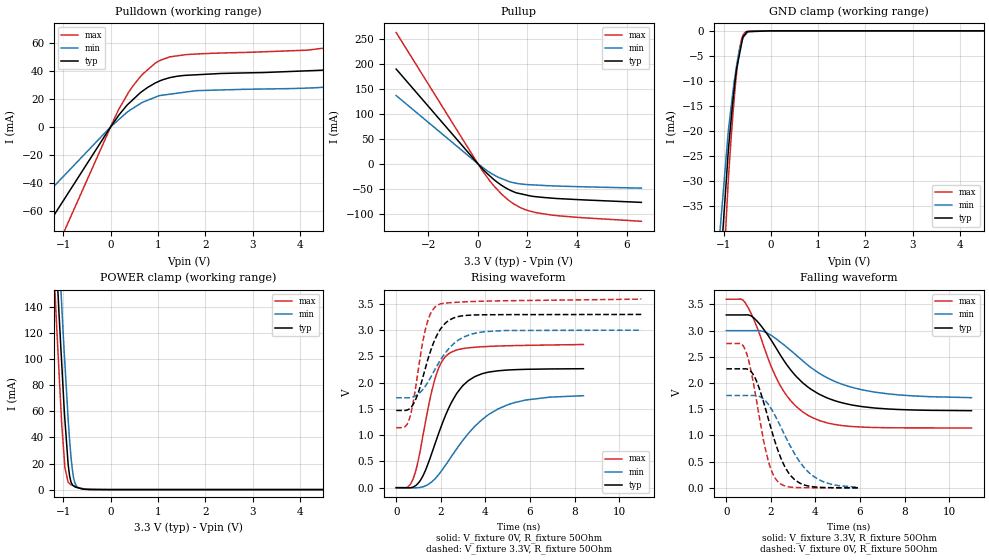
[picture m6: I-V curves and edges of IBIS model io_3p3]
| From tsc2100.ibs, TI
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|   io_3p3 Model
[Model]   io_3p3
Model_type   I/O
Polarity   Non-Inverting
Enable   Active-Low
Vinl = 0.99
Vinh = 2.31
Vmeas = 1.65
Vref = 1.65
Cref = 10pF
Rref = 50
|   typ   min   max
|   (nom PVT)   (fast PVT)   (slow PVT)
|C_comp from frequency sweep method (F=13MHz)
|Average
|C_comp   2.863e-12   2.648e-12   3.065e-12
|ON state : BUFFER OUTPUT TURNED HIGH
|C_comp   4.084e-12   3.666e-12   4.474e-12
|OFF state: BUFFER IN HIGH IMPEDANCE
|C_comp   1.642e-12   1.629e-12   1.656e-12
|C_comp from LC tank measurement(L=1nH)
|Average
|Resonant Frequency(Hz)   4.310e+09   4.340e+09   4.270e+09
C_comp   1.373e-12   1.353e-12   1.400e-12
|ON state : BUFFER OUTPUT TURNED HIGH
|Resonant Frequency(Hz)   4.130e+09   4.170e+09   4.070e+09
|C_comp   1.487e-12   1.458e-12   1.531e-12
|OFF state: BUFFER IN HIGH IMPEDANCE
|Resonant Frequency(Hz)   4.490e+09   4.510e+09   4.470e+09
|C_comp   1.258e-12   1.247e-12   1.269e-12
| Where nom  PVT is Nominal Process, 3.3V, 26C
|   Fast PVT is Strong Process,  3.6V, -40C
|   Slow PVT is Weak Process,   3V, 86C
[Model Spec]
|Subparameter   typ   min   max
Vinh   2.31   2.1   2.52
Vinl   0.99   0.9   1.08
[Voltage Range]   3.3   3   3.6
|Ambient Temperature   25   85   -40
|Junction Temperature
[Temperature Range]   26   86   -40
[Pullup Reference]   3.3   3   3.6
[Pulldown Reference]   0   0   0
[Power Clamp Reference]   3.3   3   3.6
[GND Clamp Reference]   0   0   0
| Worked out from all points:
|   slope of the pulldown table from 0 to 0.495 V, typ, clamps not added: 24.4 ohm
|   slope of the pullup table from 0 to 0.495 V, typ, clamps not added: 19.8 ohm
|   GND clamp passes 1 mA (typ) near -0.57 V on its own axis
|   POWER clamp passes 1 mA (typ) near -0.64 V on its own axis
|   falling waveform, V_fixture 3.3V, R_fixture 50Ohm: 20-80 % time 2.13ns typ, 2.66ns min, 1.62ns max; typ from 3.3 V to 1.47 V
|   rising waveform, V_fixture 0V, R_fixture 50Ohm: 20-80 % time 1.32ns typ, 2.09ns min, 821ps max; typ from 0 V to 2.27 V
|   rising waveform, V_fixture 3.3V, R_fixture 50Ohm: 20-80 % time 853ps typ, 1.22ns min, 597ps max; typ from 1.47 V to 3.3 V
|   falling waveform, V_fixture 0V, R_fixture 50Ohm: 20-80 % time 1.03ns typ, 1.4ns min, 738ps max; typ from 2.27 V to 0.001 V
[Pulldown]
|   Voltage   I(typ)   I(min)   I(max)
-3.3V     -174.4mA   -117.2mA   -251.9mA
-3mV      -158.6uA   -106.5uA   -229uA
172.8mV   8.404mA    5.266mA    12.6mA
478.8mV   19.78mA    13.48mA    29.65mA
684mV     25.89mA    17.74mA    38.01mA
1.026V    32.75mA    22.4mA     47.35mA
1.591V    36.96mA    24.99mA    51.77mA
4.162V    40.2mA     27.84mA    54.99mA
5.141V    44.75mA    31.56mA    62.91mA
5.666V    52.18mA    36.03mA    74.45mA
6.154V    64.13mA    43.44mA    92.9mA
6.6V      80.76mA    50.23mA    118mA
[GND Clamp]
|   Voltage   I(typ)   I(min)   I(max)
-3.3V     -1.799A    -1.622A    -1.991A
-1.505V   -108.3mA   -89.01mA   -138.1mA
-897.6mV  -23.79mA   -19.91mA   -29.58mA
-792mV    -13.12mA   -11.42mA   -15.51mA
-726mV    -7.734mA   -7.055mA   -8.618mA
-702mV    -6.579mA   -5.702mA   -6.431mA
-658.8mV  -4.5mA     -3.681mA   -3.454mA
-622.8mV  -2.767mA   -2.351mA   -1.787mA
-590.7mV  -1.223mA   -1.433mA   -927.5uA
-532.8mV  -520.6uA   -757.3uA   -190.4uA
-285mV    -102.3uA   -1.16uA    -4.272uA
6.6V      0A         0A         0A
[Pullup]
|   Voltage   I(typ)   I(min)   I(max)
-3.3V     189.3mA    136.3mA    262.3mA
172.8mV   -9.523mA   -6.528mA   -13.21mA
633.6mV   -31.21mA   -22.03mA   -43.6mA
939.6mV   -42.59mA   -29.3mA    -59.94mA
1.246V    -51.57mA   -35.37mA   -73.23mA
1.554V    -58.2mA    -39.1mA    -83.32mA
1.886V    -61.79mA   -41.2mA    -91.35mA
2.473V    -66.52mA   -42.91mA   -98.8mA
4.162V    -71.97mA   -45.93mA   -107.7mA
6.6V      -77.18mA   -48.73mA   -115mA
[POWER Clamp]
|   Voltage   I(typ)   I(min)   I(max)
-3.3V     1.944A     1.96A      1.945A
-1.264V   265.3mA    313.5mA    221.5mA
-1.156V   183.4mA    230.4mA    136.4mA
-1.119V   155.9mA    202.4mA    110.6mA
-1.092V   136.5mA    183mA      91.77mA
-1.037V   99.17mA    144.1mA    52.64mA
-964.8mV  53mA       95.98mA    16.49mA
-897.6mV  19.49mA    54.27mA    5.769mA
-867.9mV  10.84mA    38.76mA    4.703mA
-813mV    4.16mA     16.68mA    3.379mA
-745.8mV  1.988mA    4.458mA    2.257mA
6.6V      0A         0A         0A
[Ramp]
R_load = 50
|   typ   min   max
dV/dt_r   1.36168/1.32355e-09   1.05672/2.1169e-09   1.64582/8.29156e-10
dV/dt_f   1.09604/2.1243e-09   0.766988/2.65898e-09   1.47376/1.61142e-09
[Falling Waveform]
V_fixture = 3.3V
V_fixture_min = 3V
V_fixture_max = 3.6V
R_fixture = 50Ohm
|   Time   V(typ)   V(min)   V(max)
0s        3.3V       3V         3.6V
832ps     3.301V     3V         3.542V
1.378ns   3.183V     3.002V     3.065V
2.011ns   2.821V     2.911V     2.318V
2.429ns   2.532V     2.781V     1.945V
3.044ns   2.17V      2.567V     1.592V
3.779ns   1.888V     2.302V     1.358V
4.853ns   1.666V     2.035V     1.211V
6.091ns   1.551V     1.872V     1.16V
11ns      1.473V     1.722V     1.144V
[Rising Waveform]
V_fixture = 0V
V_fixture_min = 0V
V_fixture_max = 0V
R_fixture = 50Ohm
|   Time   V(typ)   V(min)   V(max)
0s        1.32nV     7.495nV    793.1pV
500ps     -2.558mV   -8.666uV   6.658mV
763ps     12.35mV    -2.305mV   170.9mV
1.196ns   221.4mV    16.91mV    984.8mV
1.735ns   826.7mV    166.5mV    2.067V
2.313ns   1.476V     490.5mV    2.537V
3.233ns   2.038V     1.031V     2.663V
4.562ns   2.226V     1.498V     2.697V
5.823ns   2.254V     1.67V      2.711V
8.4ns     2.266V     1.752V     2.727V
[Rising Waveform]
V_fixture = 3.3V
V_fixture_min = 3V
V_fixture_max = 3.6V
R_fixture = 50Ohm
|   Time   V(typ)   V(min)   V(max)
0s        1.471V     1.712V     1.143V
382ps     1.47V      1.712V     1.155V
584ps     1.499V     1.712V     1.3V
924ps     1.732V     1.762V     2.052V
1.313ns   2.282V     1.938V     3.02V
1.552ns   2.616V     2.107V     3.325V
1.847ns   2.92V      2.334V     3.476V
2.556ns   3.229V     2.733V     3.527V
3.702ns   3.292V     2.956V     3.549V
11ns      3.3V       3V         3.591V
[Falling Waveform]
V_fixture = 0V
V_fixture_min = 0V
V_fixture_max = 0V
R_fixture = 50Ohm
|   Time   V(typ)   V(min)   V(max)
0s        2.272V     1.763V     2.757V
656ps     2.272V     1.763V     2.753V
862ps     2.272V     1.763V     2.621V
1.06ns    2.241V     1.763V     2.328V
1.325ns   2.066V     1.761V     1.741V
1.856ns   1.36V      1.61V      557.8mV
2.286ns   750.1mV    1.298V     129.4mV
2.893ns   231.1mV    778.7mV    14.45mV
3.838ns   23.68mV    242.9mV    1.81mV
5.912ns   1.168mV    12.38mV    481.4uV
